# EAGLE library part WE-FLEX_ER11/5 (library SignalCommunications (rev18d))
WE-FLEX Flexible Transformer for DC/DC Converter Characteristics Transformer with 6 identical windings 4 sizes with 5 different lengths of air gap each Insulation test voltage 500 VAC Low leakage inductance Operating temperature: –40 ºC to +125 ºC By using different circuits more than 375 transformer solutions and about 125 choke solutions possible. Consequently, quick prototyping possibilities Applications All kind of switching regulators -Flyback converters -Forward converters -Push-pull converters -Step-up/step-down converters -SEPIC converter Details see: http://katalog.we-online.de/en/pbs/WE-FLEX? Updated by Dan Xu 2014-07-07 2014 (C) Wurth Elektronik
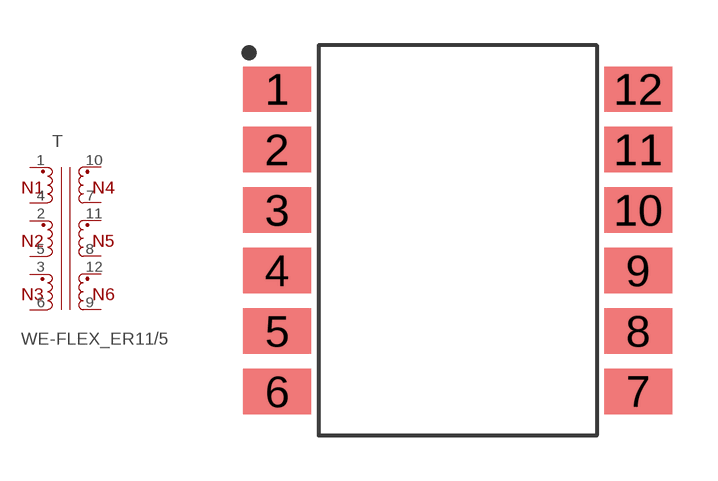
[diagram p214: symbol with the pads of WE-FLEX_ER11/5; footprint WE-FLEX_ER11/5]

Designator prefix T

## WE-FLEX_ER11/5_749196101, WE-FLEX_ER11/5_749196111, WE-FLEX_ER11/5_749196121, WE-FLEX_ER11/5_749196131, WE-FLEX_ER11/5_749196141  [WE-FLEX_ER11/5]
1  1  pas
2  11  pas
3  9  pas
4  12  pas
5  10  pas
6  8  pas
7  3  pas
8  5  pas
9  7  pas
10  2  pas
11  4  pas
12  6  pas

## Footprint WE-FLEX_ER11/5 (pad centres in mm)
smd 2.25 x 1.5: 1 -5.975,5; 2 -5.975,3; 3 -5.975,1; 4 -5.975,-1; 5 -5.975,-3; 6 -5.975,-5; 7 5.975,-5; 8 5.975,-3; 9 5.975,-1; 10 5.975,1; 11 5.975,3; 12 5.975,5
